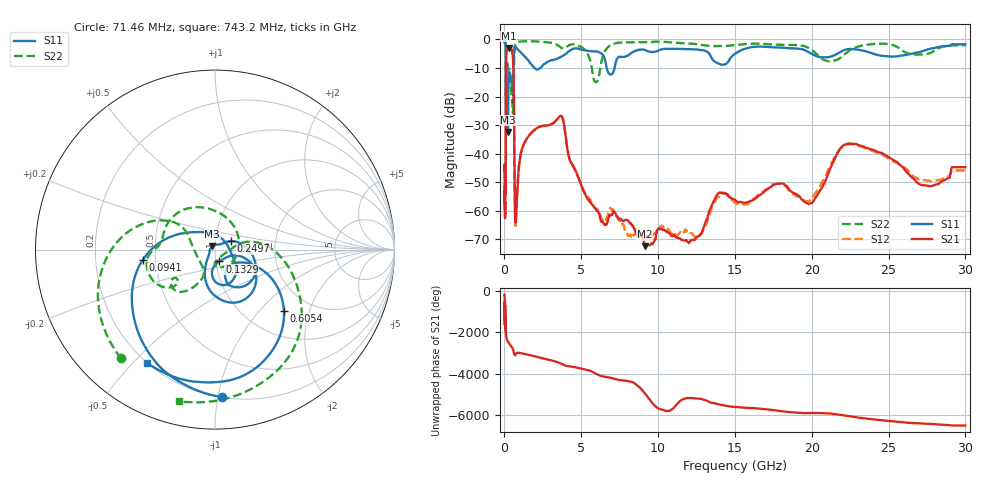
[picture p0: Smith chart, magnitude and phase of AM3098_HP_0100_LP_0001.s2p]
! Date/Time: Thu, Feb 28, 2019 8:34 AM
! Network Analyzer: Agilent Technologies E8364B Rev: A.07.50.67
! Sweep from 0.010 to 30.000 GHz, 1601 Points, Sweep Type: LOG
! Power Supply: 5.022 V, 0.002 A
# Hz S DB R 50
!freq MagS11 AngS11 MagS21 AngS21 MagS12 AngS12 MagS22 AngS22
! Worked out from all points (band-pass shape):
!   1601 points, 10 MHz to 30 GHz, reference 50 ohm
!   highest |S21| = -3.00 dB at 267.8 MHz (marker M1); lowest = -72.4 dB at 9.118 GHz (marker M2)
!   |S21| within 3 dB of the highest: 111.2 MHz to 546.3 MHz (435.1 MHz wide, 132 % of centre)
!   lowest |S11| = -32.4 dB at 229.3 MHz (marker M3), VSWR 1.05, Z = 48.4 + j1.76 ohm
!   |S11| at or under -10 dB: 176.1 MHz to 571.3 MHz (395.1 MHz wide, 106 % of centre); 1.964 GHz to 2.325 GHz (361.7 MHz wide, 16.9 % of centre); 6.651 GHz to 7.164 GHz (512.3 MHz wide, 7.42 % of centre)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
!   |S22| runs from -25.9 to -0.6 dB; largest |S21 - S12| = 0.01
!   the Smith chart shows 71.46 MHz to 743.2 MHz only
!   S11 on the Smith chart (normalised r, x): 71.46 MHz: 0.20, -1.03; 94.1 MHz: 0.42, -0.06; 132.9 MHz: 1.04, -0.14; 249.7 MHz: 1.19, +0.11; 605.4 MHz: 1.48, -1.38; 743.2 MHz: 0.20, -0.55
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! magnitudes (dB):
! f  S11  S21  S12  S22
! 10 MHz  -0.3  -45.8  -46.4  -0.6
! 38.04 MHz  -0.5  -58.9  -61.9  -0.8
! 71.46 MHz  -1.7  -52.1  -52.3  -1.9
! 94.1 MHz  -7.8  -20.9  -20.8  -9.4
! 132.9 MHz  -23.0  -4.1  -4.0  -11.3
! 144.7 MHz  -15.8  -3.7  -3.6  -10.8
! 186.8 MHz  -11.2  -3.5  -3.5  -8.2
! 229.3 MHz  -32.4  -3.1  -3.1  -9.9
! 249.7 MHz  -19.8  -3.0  -3.0  -10.3
! 267.8 MHz  -15.2  -3.0  -3.0  -10.5
! 550.5 MHz  -13.5  -6.3  -6.2  -25.9
! 605.4 MHz  -5.8  -15.5  -15.4  -11.4
! 679.2 MHz  -2.6  -58.3  -58.6  -2.2
! 743.2 MHz  -2.7  -63.1  -64.3  -1.2
! 1.029 GHz  -4.4  -41.0  -41.1  -0.7
! 2.084 GHz  -10.5  -31.1  -31.2  -0.7
! 3.704 GHz  -6.0  -26.8  -26.8  -2.9
! 7.926 GHz  -5.9  -63.2  -67.4  -1.0
! 9.118 GHz  -3.6  -72.4  -68.3  -1.0
! 19.9 GHz  -4.7  -57.4  -56.1  -3.2
! 22.56 GHz  -3.3  -36.5  -36.7  -3.5
! 30 GHz  -1.7  -44.7  -45.8  -2.1
